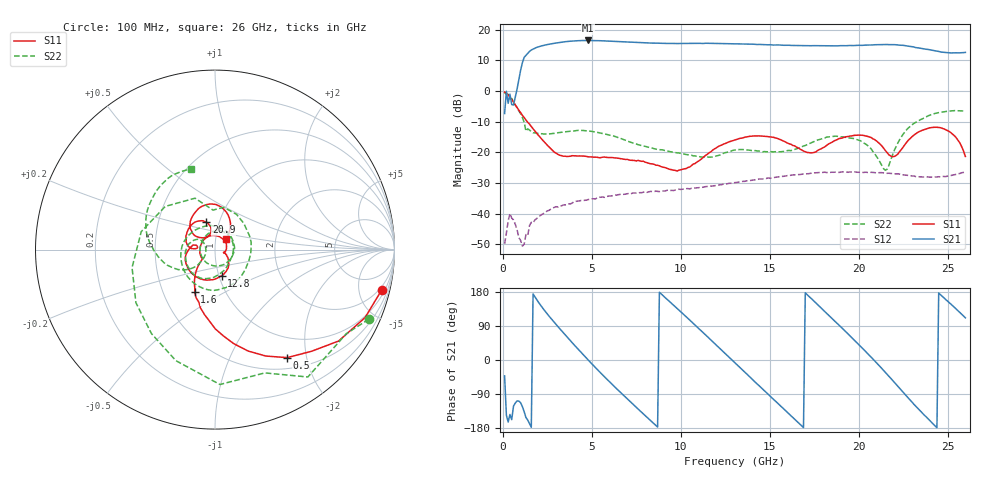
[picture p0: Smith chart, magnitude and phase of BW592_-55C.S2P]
!Keysight Technologies,N5247A,US51370447,A.10.64.09
!Date: Thursday, March 05, 2020 06:55:08
!Correction: S11(Full 2 Port with power(1,2))
!S21(Full 2 Port with power(1,2))
!S12(Full 2 Port with power(1,2))
!S22(Full 2 Port with power(1,2))
!S2P File: Measurements: S11, S21, S12, S22:
# Hz S  dB  R 50
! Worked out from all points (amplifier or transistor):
!   260 points, 100 MHz to 26 GHz, reference 50 ohm
!   highest |S21| = 16.4 dB at 4.8 GHz (marker M1)
!   |S21| within 3 dB of that: 1.637 GHz to 23.96 GHz (22.33 GHz wide, 174 % of centre)
!   unconditionally stable (mu >= 1): start of sweep to end of sweep
!   at 4.4 GHz: K = 4.42, MAG = 16.6 dB, |S12| = -35.7 dB
!   at 13.1 GHz: K = 2.63, MAG = 15.6 dB, |S12| = -29.9 dB
!   at 26 GHz: K = 2.04, MAG = 13.7 dB, |S12| = -26.5 dB
!   S11 on the Smith chart (normalised r, x): 100 MHz: 1.57, -8.19; 500 MHz: 0.66, -1.67; 1.6 GHz: 0.72, -0.37; 12.8 GHz: 1.03, -0.31; 20.9 GHz: 0.87, +0.27; 26 GHz: 1.12, +0.14
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1e8  -0.39 -13.4  -7.39 -41.8  -49.83 48.2  -0.53 -24.3
5e8  -2.81 -56.3  -4.47 -157.4  -41.46 -6.9  -2.47 -87.9
1.2e9  -8.68 -99.0  10.94 -136.5  -49.92 23.2  -10.25 111.2
1.6e9  -11.63 -115.5  13.34 -177.4  -42.84 16.3  -13.26 42.3
3.1e9  -20.69 -142.2  15.71 88.0  -37.88 -21.4  -13.64 -45.1
4.5e9  -21.24 -164.7  16.42 15.0  -35.76 -61.5  -12.89 -104.2
4.8e9  -21.50 -175.6  16.44 -0.0  -35.41 -70.2  -13.03 -117.1
6.6e9  -22.09 93.0  16.04 -85.1  -33.73 -124.9  -15.41 154.1
7.9e9  -22.92 27.2  15.71 -142.5  -33.02 -169.1  -17.97 76.3
8.8e9  -24.41 -7.3  15.54 178.7  -32.82 159.8  -19.15 17.9
1.09e10  -23.23 -24.2  15.50 88.1  -31.59 76.9  -21.32 -130.2
1.28e10  -16.45 -75.7  15.39 3.8  -30.11 -3.3  -19.69 89.4
1.31e10  -15.90 -86.3  15.36 -9.9  -29.86 -16.0  -19.24 73.5
1.5e10  -14.93 -154.7  15.05 -94.2  -28.42 -93.9  -19.87 -8.5
1.62e10  -17.41 173.4  14.82 -147.7  -27.48 -139.6  -19.48 -45.8
1.74e10  -20.19 173.5  14.75 159.4  -26.83 174.6  -16.76 -85.8
1.91e10  -15.33 159.8  14.73 82.5  -26.38 107.3  -14.99 -147.5
2.09e10  -15.88 107.7  15.04 -2.2  -26.63 31.8  -20.47 146.6
2.17e10  -20.83 107.6  15.09 -43.0  -26.83 -6.3  -24.28 -152.5
2.26e10  -17.53 145.3  14.76 -90.5  -27.42 -52.0  -13.40 -148.2
2.39e10  -12.17 112.1  13.52 -155.0  -28.04 -117.7  -8.13 166.5
2.6e10  -21.38 44.6  12.55 111.3  -26.47 143.0  -6.59 106.3
